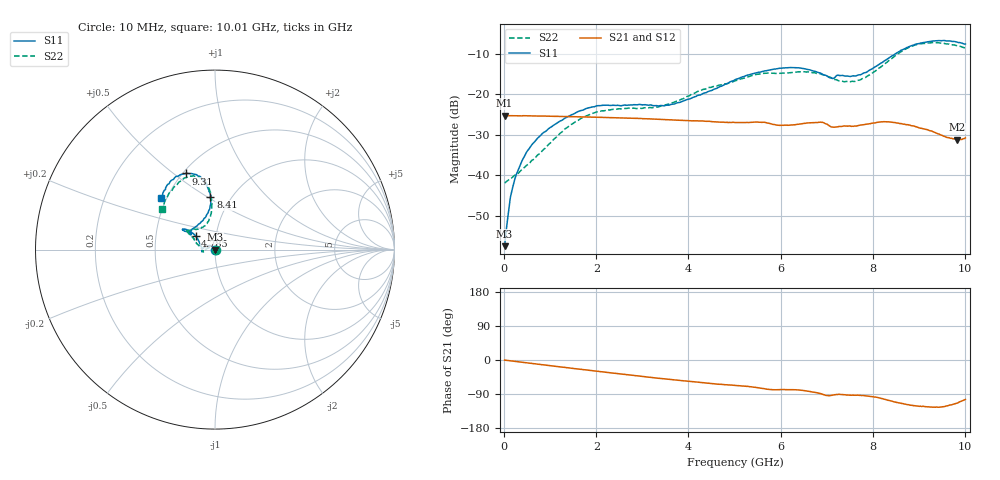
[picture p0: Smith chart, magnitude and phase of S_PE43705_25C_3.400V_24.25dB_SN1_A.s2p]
! Device ID: PE43705
! Serial: 1
! Insertion: A
! Impedance: 50 ohm
! Temp: 25C
! VDD: 3.400V
! Attenuation Step: 24.25dB
#  Hz  S  RI  R  50
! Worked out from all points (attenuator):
!   401 points, 10 MHz to 10.01 GHz, reference 50 ohm
!   highest |S21| = -25.25 dB at 10 MHz (marker M1); lowest = -31.2 dB at 9.835 GHz (marker M2)
!   lowest |S11| = -57.5 dB at 10 MHz (marker M3), VSWR 1.00, Z = 49.9 + j0.0449 ohm
!   |S11| at or under -10 dB: start of sweep to 8.49 GHz
!   |S22| runs from -41.9 to -7.3 dB; largest |S21 - S12| = 0.00074
!   S11 on the Smith chart (normalised r, x): 10 MHz: 1.00, +0.00; 4.785 GHz: 0.80, +0.12; 8.41 GHz: 0.80, +0.52; 9.31 GHz: 0.52, +0.56; 10.01 GHz: 0.47, +0.33
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1e7  -0.00126 0.00045  0.0546 -0.000222  0.0547 -0.000162  0.00804 0.000283
1.1e8  -0.00103 0.00405  0.0544 -0.00167  0.0544 -0.00161  0.00828 0.00321
1.85e8  -0.00176 0.00688  0.0543 -0.00274  0.0544 -0.00273  0.00774 0.00551
3.1e8  -0.00365 0.0113  0.0541 -0.00454  0.054 -0.00449  0.00589 0.00885
4.85e8  -0.00838 0.0173  0.0538 -0.00703  0.0537 -0.00696  0.00153 0.0132
9.85e8  -0.0308 0.0228  0.0519 -0.0137  0.0519 -0.0137  -0.0196 0.015
1.685e9  -0.0624 0.0102  0.0477 -0.0221  0.0477 -0.0221  -0.0508 0.00215
2.21e9  -0.0732 -0.00569  0.0437 -0.0277  0.0437 -0.0277  -0.0627 -0.0101
3.36e9  -0.0719 -0.00321  0.0326 -0.0367  0.0326 -0.0366  -0.0702 -0.00157
3.835e9  -0.0777 0.0198  0.0279 -0.0388  0.0278 -0.0388  -0.0848 0.0167
4.785e9  -0.1079 0.0767  0.0191 -0.0408  0.0192 -0.0408  -0.1196 0.0619
5.01e9  -0.1215 0.09  0.0173 -0.0413  0.0176 -0.0413  -0.1281 0.0712
5.985e9  -0.1757 0.1144  0.00856 -0.0404  0.00874 -0.0405  -0.1496 0.1019
6.685e9  -0.167 0.1019  0.00438 -0.0444  0.00421 -0.0445  -0.1512 0.106
7.11e9  -0.1317 0.0865  -0.00226 -0.0394  -0.00212 -0.0395  -0.1101 0.1129
7.61e9  -0.0875 0.1434  -0.00204 -0.0407  -0.00185 -0.0406  -0.0551 0.1329
8.36e9  -0.0225 0.2828  -0.0132 -0.0436  -0.0133 -0.0434  -0.0187 0.263
8.41e9  -0.0256 0.2941  -0.0143 -0.0428  -0.0145 -0.0429  -0.0203 0.2746
8.86e9  -0.0751 0.3941  -0.0202 -0.0354  -0.0201 -0.0354  -0.0673 0.3879
9.31e9  -0.1616 0.4245  -0.0195 -0.0284  -0.0195 -0.0284  -0.1499 0.4067
9.835e9  -0.2757 0.3429  -0.0112 -0.0252  -0.0114 -0.0252  -0.2648 0.2953
1.001e10  -0.2992 0.29  -0.00711 -0.0281  -0.00753 -0.0279  -0.2965 0.2284
